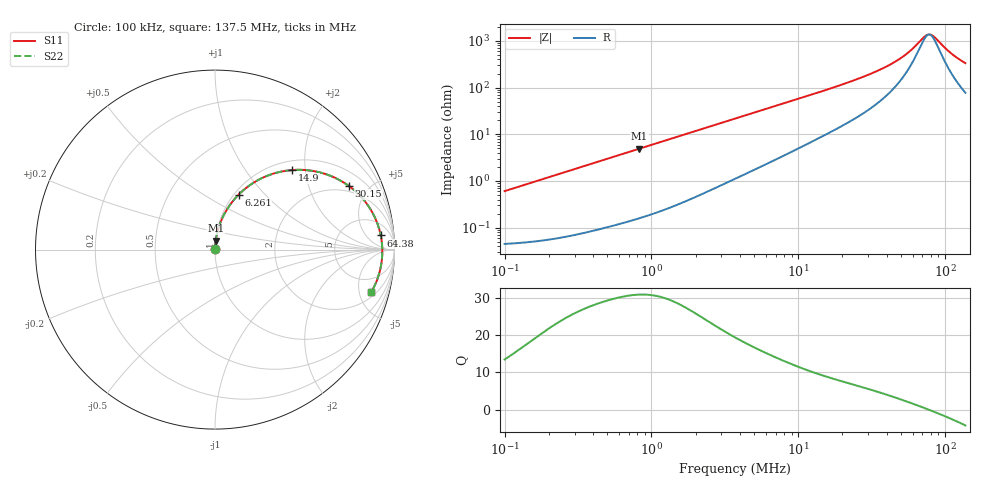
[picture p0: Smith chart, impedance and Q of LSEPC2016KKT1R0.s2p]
! LSEPC2016KKT1R0  S-PARAMETER MODEL  ( General Type )
! Model Generated by TAIYO YUDEN Corporation (http://www.ty-top.com)
! Version 1.0
! TAIYO YUDEN Control No. 180907NI43SB-FBB
! Copyright(c) 2018 TAIYO YUDEN CO.,LTD. All Rights Reserved.
! Product Description (link to TY-COMPAS)
! https://ds.yuden.co.jp/TYCOMPAS/or/detail?pn=LSEPC2016KKT1R0M&u=M
! Products Name : Inductors
! Characteristics :
!  Inductance : 1.0 uH , SRF(min) : -Hz , DC Resistance(max) : 0.048 Ohm
!  Rated Current : Saturation :4000 mA , Temp Rise : 3500 mA (40 degC)
!  Case Size : 2.0 x 1.6 / 0.079 x 0.063 [mm/inch] , Thickness : 1 / 0.039 [mm/inch]
!  (Conditions: Temperature = 25 degC , DC Bias Current/Voltage = 0A / 0V)
! External Node Assignments :
!  1  o---GGG---o  2
! GND o---------o GND
! Frequency Range : 0.1MHz  -  137.487582MHz  [ 402 STEP ]
# MHz S RI R 50
! Freq[MHz].  S11 Real  S11 Imag  S21 Real  S21 Imag  S12 Real  S12 Imag  S22 Real  S22 Imag
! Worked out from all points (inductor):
!   401 points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, 100 kHz to 137.5 MHz, reference 50 ohm
!   read as one part in series: L = 963 nH near 103.7 kHz
!   highest Q = 30.9 at 827.8 kHz (marker M1), where L = 945 nH
!   self-resonance near 77.78 MHz
!   S11 on the Smith chart (normalised r, x): 100 kHz: 1.00, +0.01; 6.261 MHz: 1.05, +0.72; 14.9 MHz: 1.19, +1.70; 30.15 MHz: 1.67, +3.73; 64.38 MHz: 12, +13; 137.5 MHz: 2.55, -6.50
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0.1  0.000486 0.00605  0.9995 -0.00605  0.9995 -0.00605  0.000486 0.00605
0.335474  0.00116 0.0201  0.9988 -0.0201  0.9988 -0.0201  0.00116 0.0201
0.827832  0.00399 0.0489  0.996 -0.0489  0.996 -0.0489  0.00399 0.0489
1.125429  0.00658 0.066  0.9934 -0.066  0.9934 -0.066  0.00658 0.066
2.117953  0.0199 0.1213  0.9801 -0.1213  0.9801 -0.1213  0.0199 0.1213
3.707932  0.054 0.2016  0.946 -0.2016  0.946 -0.2016  0.054 0.2016
6.261175  0.131 0.3055  0.869 -0.3055  0.869 -0.3055  0.131 0.3055
8.825176  0.2222 0.3772  0.7778 -0.3772  0.7778 -0.3772  0.2222 0.3772
12.43915  0.3511 0.4306  0.6489 -0.4306  0.6489 -0.4306  0.3511 0.4306
14.9021  0.4312 0.4434  0.5688 -0.4434  0.5688 -0.4434  0.4312 0.4434
21.00463  0.5916 0.4282  0.4084 -0.4282  0.4084 -0.4282  0.5916 0.4282
30.14589  0.7459 0.3546  0.2541 -0.3546  0.2541 -0.3546  0.7459 0.3546
41.73016  0.8501 0.2493  0.1499 -0.2493  0.1499 -0.2493  0.8501 0.2493
52.77686  0.8993 0.1595  0.1007 -0.1595  0.1007 -0.1595  0.8993 0.1595
64.37923  0.9235 0.0788  0.0765 -0.0788  0.0765 -0.0788  0.9235 0.0788
73.0576  0.9308 0.0262  0.0692 -0.0262  0.0692 -0.0262  0.9308 0.0262
77.12628  0.932 0.00354  0.068 -0.00354  0.068 -0.00354  0.932 0.00354
79.96385  0.9322 -0.0116  0.0678 0.0116  0.0678 0.0116  0.9322 -0.0116
85.95603  0.931 -0.0421  0.069 0.0421  0.069 0.0421  0.931 -0.0421
110.6918  0.9101 -0.1484  0.0899 0.1484  0.0899 0.1484  0.9101 -0.1484
125.6132  0.8895 -0.2006  0.1105 0.2006  0.1105 0.2006  0.8895 -0.2006
137.4876  0.8705 -0.2371  0.1295 0.2371  0.1295 0.2371  0.8705 -0.2371
